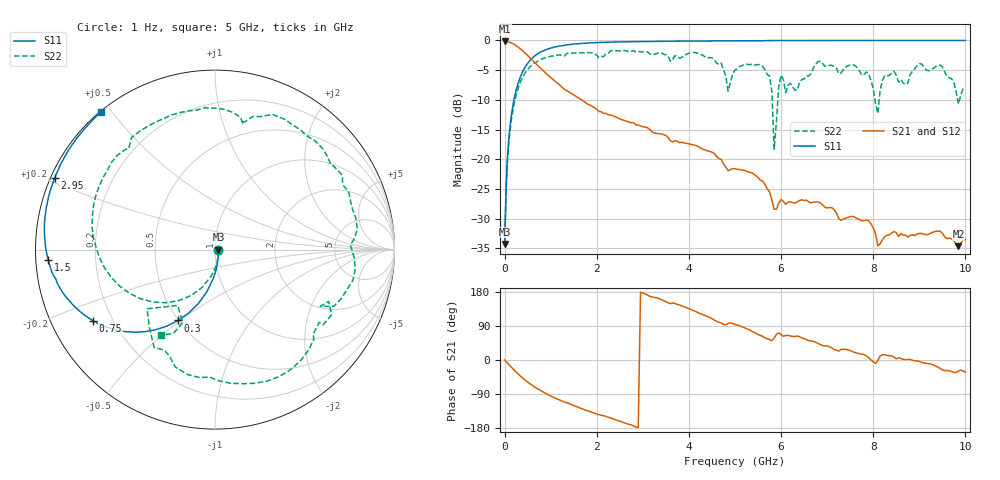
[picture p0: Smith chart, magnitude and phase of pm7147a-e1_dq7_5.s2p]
# GHz S DB R 50
! S-Parameters data
! Freq  dbS11  angS11  dbS21  angS21  dbS12  angS12  dbS22  angS22
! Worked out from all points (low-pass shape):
!   279 points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, 1 Hz to 10 GHz, reference 50 ohm
!   highest |S21| = -0.17 dB at 794.3 Hz (marker M1); lowest = -34.6 dB at 9.85 GHz (marker M2)
!   |S21| within 3 dB of the highest: start of sweep to 583.1 MHz
!   lowest |S11| = -34.3 dB at 794.3 Hz (marker M3), VSWR 1.04, Z = 52 - j0.000131 ohm
!   |S11| at or under -10 dB: start of sweep to 202.2 MHz
!   |S22| runs from -34.3 to -1.7 dB; largest |S21 - S12| = 0
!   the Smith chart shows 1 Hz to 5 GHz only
!   S11 on the Smith chart (normalised r, x): 1 Hz: 1.04, -0.00; 300 MHz: 0.50, -0.49; 750 MHz: 0.13, -0.27; 1.5 GHz: 0.04, -0.03; 2.95 GHz: 0.01, +0.21; 5 GHz: 0.00, +0.47
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1e-09  -34.28 -0.0  -0.17 -0.0  -0.17 -0.0  -34.28 -0.0
7.943e-07  -34.28 -0.0  -0.17 -0.0  -0.17 -0.0  -34.28 -0.0
0.1  -15.74 -93.7  -0.29 -13.1  -0.29 -13.1  -16.49 -98.3
0.3  -7.04 -117.4  -1.15 -37.6  -1.15 -37.6  -7.90 -132.7
0.75  -2.09 -149.6  -4.46 -78.5  -4.46 -78.5  -3.34 174.5
1.5  -0.62 -176.5  -9.18 -120.2  -9.18 -120.2  -2.11 114.8
1.7  -0.49 178.6  -10.17 -129.5  -10.17 -129.5  -2.08 100.7
2.95  -0.19 155.8  -14.41 178.9  -14.41 178.9  -1.92 19.4
3.35  -0.15 150.0  -15.68 162.1  -15.68 162.1  -2.05 -7.6
4.2  -0.09 138.9  -17.85 124.8  -17.85 124.8  -2.19 -73.4
5  -0.05 129.5  -21.62 93.8  -21.62 93.8  -4.96 -122.3
5.05  -0.04 129.0  -21.70 92.4  -21.70 92.4  -4.75 -126.2
5.75  -0.03 121.7  -25.53 54.1  -25.53 54.1  -6.03 152.8
5.85  -0.02 120.7  -28.44 57.4  -28.44 57.4  -18.33 133.9
6  -0.02 119.2  -26.79 67.1  -26.79 67.1  -5.85 -170.7
6.7  -0.01 112.6  -27.23 49.2  -27.23 49.2  -4.64 161.7
7.55  -0.01 105.3  -29.65 22.2  -29.65 22.2  -4.06 104.4
8.1  -0.00 101.0  -34.61 -1.4  -34.61 -1.4  -12.31 100.1
8.35  -0.00 99.1  -32.73 11.6  -32.73 11.6  -5.91 90.8
9.5  -0.00 91.2  -32.44 -26.1  -32.44 -26.1  -4.45 34.6
9.85  -0.00 89.0  -34.64 -29.1  -34.64 -29.1  -10.69 24.7
10  -0.00 88.1  -33.59 -32.2  -33.59 -32.2  -8.24 30.4
